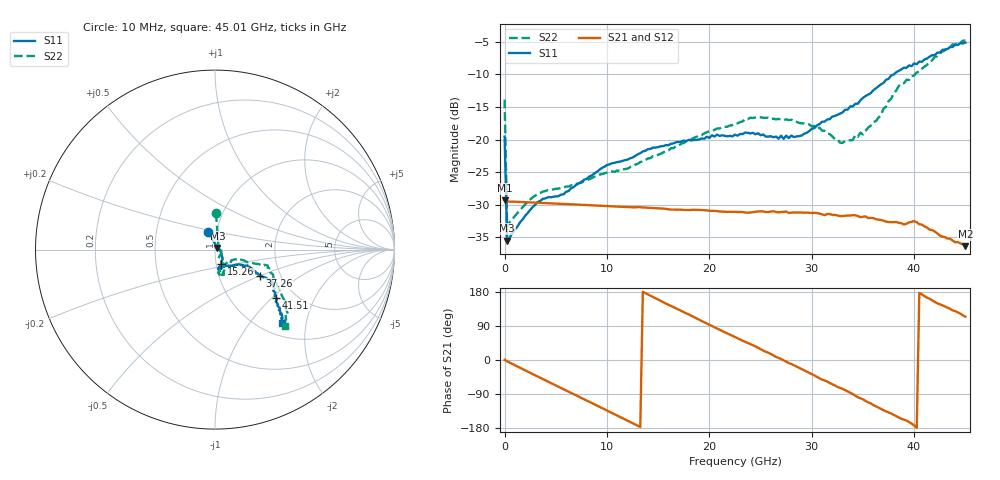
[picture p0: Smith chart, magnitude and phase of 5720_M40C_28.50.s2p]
! Device:  ADRF5720
! Description: 0.5dB LSB GaAs MMIC 6-bit Digital Attenuator
! Frequency:  0.000009 -  40 GHz
! Ports:
!	RF1	= Port 1
!	RF2	= Port 2
! Vdd:  3.3 Volt
! Vss:  -3.3 Volt
! Control:  0/3.3 Volt
! State:  28.50 dB attenuation
! Data:  The device was measured using G-S-G Probes on a matrix board.
!  Data was collected using an calibrated 4 port network analyzer.
!  The reference plane for this measurement is at the launchers.
! Note:  Analog Devices supplies this data as a sample of measured data
!  for this product.  Your particular data for this product may vary.
!  Data was taken at -40 degrees C.
!  Analog Devices reserves the right to change this data at anytime.
# GHZ S DB R 45.0
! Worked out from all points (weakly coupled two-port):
!   181 points, 10 MHz to 45.01 GHz, reference 45 ohm
!   highest |S21| = -29.32 dB at 10 MHz (marker M1); lowest = -36.4 dB at 45.01 GHz (marker M2)
!   lowest |S11| = -35.5 dB at 260 MHz (marker M3), VSWR 1.03, Z = 46.3 + j0.883 ohm
!   |S11| at or under -10 dB: start of sweep to 38.01 GHz
!   |S22| runs from -33.4 to -4.8 dB; largest |S21 - S12| = 0.00016
!   S11 on the Smith chart (normalised r, x): 10 MHz: 0.91, +0.18; 15.26 GHz: 1.06, -0.17; 37.26 GHz: 1.56, -0.50; 41.51 GHz: 1.60, -1.06; 45.01 GHz: 1.24, -1.47
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0.01  -19.53 112.3  -29.32 0.4  -29.34 0.4  -13.86 88.3
0.26  -35.50 34.6  -29.51 -3.7  -29.53 -3.7  -33.41 22.5
3.26  -29.59 -9.0  -29.70 -43.9  -29.73 -44.0  -28.31 -29.3
5.76  -28.42 -25.0  -29.88 -77.0  -29.91 -77.0  -27.40 -48.7
7.76  -26.18 -39.2  -30.04 -103.4  -30.06 -103.5  -26.41 -62.1
10.01  -23.91 -48.2  -30.22 -133.3  -30.24 -133.3  -25.07 -65.8
12.01  -23.08 -56.0  -30.36 -159.9  -30.38 -160.0  -24.48 -65.9
15.26  -21.03 -66.5  -30.56 155.8  -30.58 155.8  -22.18 -62.0
20.26  -19.34 -77.7  -30.94 89.4  -30.96 89.3  -18.61 -62.5
22.76  -19.41 -80.1  -31.13 57.4  -31.15 57.3  -17.51 -69.1
24.01  -19.06 -75.1  -31.20 42.1  -31.22 42.0  -16.64 -70.8
27.26  -19.89 -65.6  -31.10 -1.0  -31.11 -1.1  -17.01 -77.3
30.26  -18.24 -47.0  -31.26 -40.7  -31.29 -40.8  -17.90 -79.8
33.01  -15.84 -31.0  -31.75 -76.2  -31.79 -76.2  -20.51 -59.3
35.01  -13.60 -27.4  -31.85 -103.7  -31.88 -103.9  -19.22 -32.5
37.26  -10.82 -30.5  -32.61 -135.5  -32.64 -135.7  -14.94 -21.1
37.76  -10.16 -29.9  -32.69 -141.2  -32.70 -141.4  -13.73 -20.4
38.51  -9.43 -29.6  -32.78 -151.9  -32.80 -152.0  -11.76 -18.2
39.76  -8.72 -30.4  -32.63 -167.9  -32.64 -168.0  -10.26 -16.8
41.51  -7.27 -38.2  -33.83 161.5  -33.84 161.7  -8.06 -29.2
43.76  -5.78 -43.9  -35.50 131.0  -35.56 131.1  -5.35 -41.4
45.01  -5.11 -47.5  -36.37 114.1  -36.43 113.8  -4.78 -47.3
